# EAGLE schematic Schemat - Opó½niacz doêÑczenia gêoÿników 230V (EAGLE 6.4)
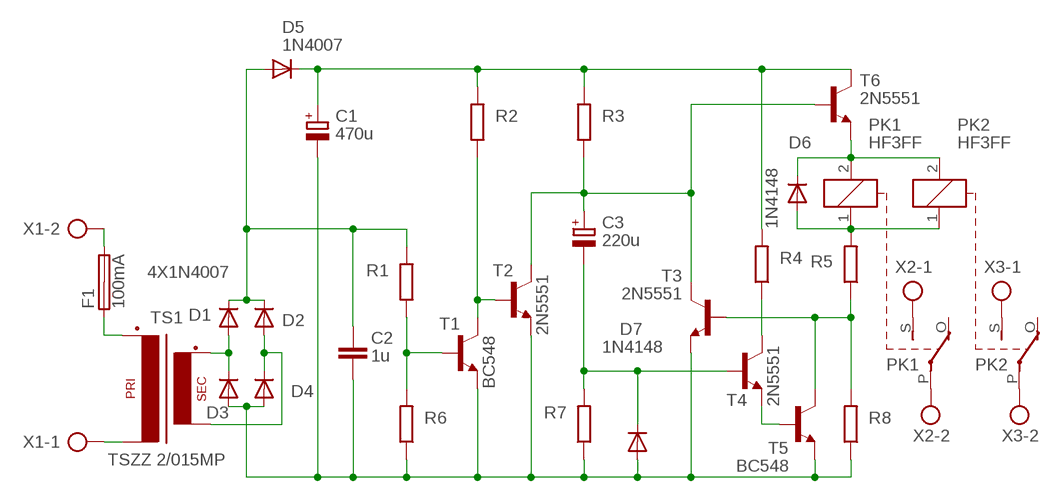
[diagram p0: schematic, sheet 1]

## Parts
C1  470u  CPOL-EUE5-13  [E5-13]
C2  1u  C-EU050-055X075  [C050-055X075]
C3  220u  CPOL-EUE5-13  [E5-13]
D1  4X1N4007  1N40047.62  [DO41-7.6]
D2  1N4007  1N40047.62  [DO41-7.6]
D3  1N4007  1N40047.62  [DO41-7.6]
D4  1N4007  1N40047.62  [DO41-7.6]
D5  1N4007  1N40047.62  [DO41-7.6]
D6  1N4148  1N4148DO35-7  [DO35-7]
D7  1N4148  1N4148DO35-7  [DO35-7]
F1  100mA  SHK20L  [SHK20L]
PK1  HF3FF  G5L  [G5LE]
PK2  HF3FF  G5L  [G5LE]
R1  R-EU_0207/7  [0207/7]
R2  R-EU_0207/7  [0207/7]
R3  R-EU_0207/7  [0207/7]
R4  R-EU_0207/7  [0207/7]
R5  R-EU_0207/7  [0207/7]
R6  R-EU_0207/7  [0207/7]
R7  R-EU_0207/7  [0207/7]
R8  R-EU_0207/7  [0207/7]
T1  BC548  BC548A  [TO92-EBC]
T2  2N5551  -NPN-TO92-EBC  [TO92-EBC]
T3  2N5551  -NPN-TO92-EBC  [TO92-EBC]
T4  2N5551  -NPN-TO92-EBC  [TO92-EBC]
T5  BC548  BC548A  [TO92-EBC]
T6  2N5551  -NPN-TO92-EBC  [TO92-EBC]
TS1  TSZZ 2/015MP  EI30_AVT  [EI30_AVT]
X1  AK500/2  [AK500/2]
X2-  ARK7.5/2  [X2.2]
X3-  ARK7.5/2  [X2.2]

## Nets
N$1: R1.1 R6.2 T1.B
N$2: F1.1A TS1.5(P2)
N$4: R2.1 T1.C T2.B
N$5: D6.C PK1.2 PK2.2 T6.E
N$6: D6.A PK1.1 PK2.1 R5.2
N$7: PK1.S(2:S) X2-.1
N$8: C3.- D7.C R7.2 T4.B
N$9: C3.+ R3.1 T2.C T3.C T6.B
N$10: C1.+ D5.C R2.2 R3.2 R4.2 T6.C
N$11: PK1.P(2:P) X2-.2
N$12: PK2.S(2:S) X3-.1
N$13: C2.1 D1.C D2.C D5.A R1.2
N$14: PK2.P(2:P) X3-.2
N$15: T4.E T5.B
N$16: TS1.1 X1.1
N$17: R5.1 R8.2 T3.B T5.C
N$18: C1.- C2.2 D3.A D4.A D7.A R6.1 R7.1 R8.1 T1.E T2.E T3.E T5.E
N$19: R4.1 T4.C
N$20: F1.2A X1.2
N$24: D1.A D3.C TS1.7(S3)
N$25: D2.A D4.C TS1.9(S4)
Unconnected: F1.1B F1.2B PK1.O(2:O) PK2.O(2:O)

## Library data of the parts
C1 C3 = rcl:CPOL-EU: POLARIZED CAPACITOR, European symbol
C2 = rcl:C-EU: CAPACITOR, European symbol
D1-D5 = diode:1N4004: DIODE
D6 D7 = diode:1N4148: DIODE
F1 = fuse:SHK20L: FUSE HOLDER 5 x 20 mm, SH contact, SHH1 Schukat, E1073 Buerklin; OC_FARNELL: unknown; OC_NEWARK: unknown
PK1 PK2 = relay:G5L: RELAY 1 x switch, 10 A/120 V AC, 8 A/30 V ADC, Omron; OC_FARNELL: unknown; OC_NEWARK: unknown
R1-R8 = rcl:R-EU_: RESISTOR, European symbol
T1 T5 = transistor-npn:BC548*: NPN Transistor
T2-T4 T6 = transistor:*-NPN-: NPN Transistror BF959 corrected 2008.03.06
TS1 = trafo:EI30_AVT
X1 = con-ptr500:AK500/2: CONNECTOR; OC_FARNELL: unknown; OC_NEWARK: unknown
X2- X3- = con-ptr750:ARK7.5/2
